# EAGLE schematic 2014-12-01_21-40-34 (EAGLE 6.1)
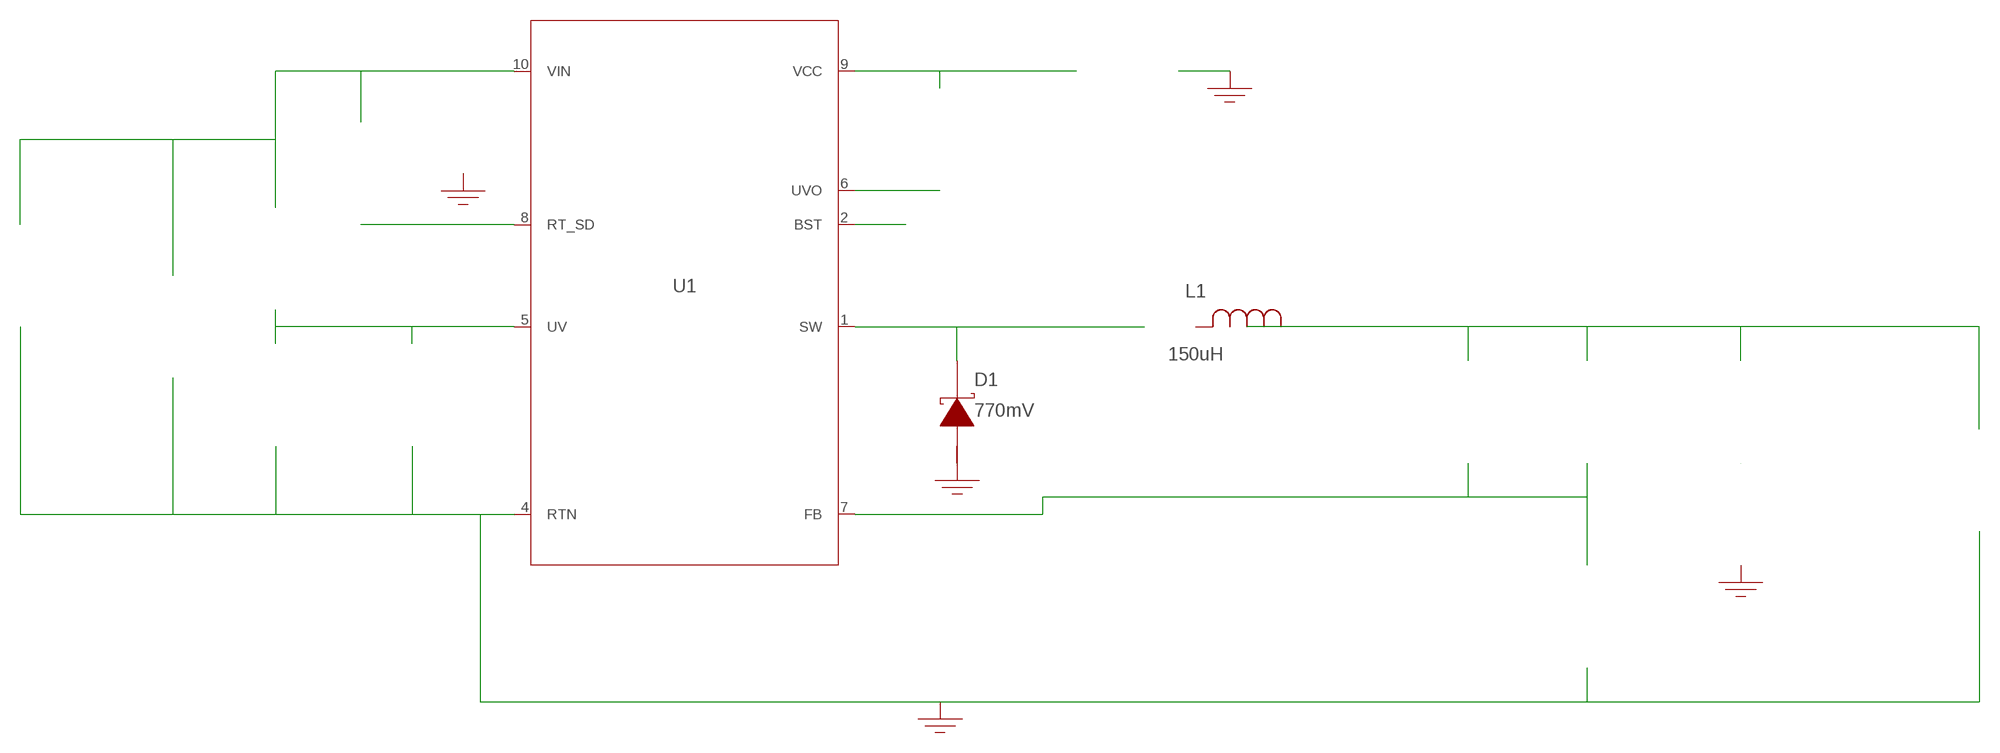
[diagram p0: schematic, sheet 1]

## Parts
CB  10nF  C1005X7R1C103KC1005X7R1C103K  [1005]  (not placed on a sheet)
CBYP  1uF  C1608X5R1C105KC1608X5R1C105K  [1608]  (not placed on a sheet)
CFF  2nF  GRM1885C1H202JA01DGRM1885C1H202JA01D  [0603]  (not placed on a sheet)
CIN  47uF  EEV-FK2A470QEEV-FK2A470Q  [SM_RADIAL_H13]  (not placed on a sheet)
CINX  100nF  C2012X7R2A104KC2012X7R2A104K  [0805]  (not placed on a sheet)
COUT  4.7uF  GRM21BR61C475KA88LGRM21BR61C475KA88L  [0805]  (not placed on a sheet)
CUV  1nF  GRM033R71E102KA01DGRM033R71E102KA01D  [0201]  (not placed on a sheet)
D1  770mV  DFLS1100-7DFLS1100-7  [PowerDI123]
GND  WB_GND  WB_GNDWB_GND  [WB_GND]
GND1  WB_GND  WB_GNDWB_GND  [WB_GND]
GND2  WB_GND  WB_GNDWB_GND  [WB_GND]
GND9999  WB_GND  WB_GNDWB_GND  [WB_GND]
GND_5  WB_GND  WB_GNDWB_GND  [WB_GND]
IOUT  WB_CURRENT_LOAD  WB_CURRENT_LOADWB_CURRENT_LOAD  [WB_CURRENT_LOAD]  (not placed on a sheet)
L1  150uH  CLF10040T-151MCLF10040T-151M  [CLF10040]
RFBB  3.32k  CRCW04023K32FKEDCRCW04023K32FKED  [0402]  (not placed on a sheet)
RFBT  10k  CRCW040210K0FKEDCRCW040210K0FKED  [0402]  (not placed on a sheet)
RON  178k  CRCW0402178KFKEDCRCW0402178KFKED  [0402]  (not placed on a sheet)
RSERIES  620m  ERJ-2BQFR62XERJ-2BQFR62X  [0402]  (not placed on a sheet)
RUV1  93.1k  CRCW040293K1FKEDCRCW040293K1FKED  [0402]  (not placed on a sheet)
RUV2  200k  CRCW0402200KFKEDCRCW0402200KFKED  [0402]  (not placed on a sheet)
RUVO  100k  CRCW0402100KFKEDCRCW0402100KFKED  [0402]  (not placed on a sheet)
U1  LM34923MM/NOPB  LM34923MM/NOPBLM34923MM/NOPB  [MUB10A]
VIN  WB_BATTERY  WB_BATTERYWB_BATTERY  [WB_BATTERY]  (not placed on a sheet)

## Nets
0: Cbyp.2@2 Cin.-@2 Cinx.2@2 Cuv.2@2 D1.2(A) GND1.1 GND2.1 GND9999.1 GND.1 GND_5.1 Iout.-@2 Rfbb.2@2 Rseries.2@2 Ruv1.2@2 U1.3(NC) U1.4(RTN) Vin.-@2
1: Cuv.1@1 Ruv1.1@1 Ruv2.2@2 U1.5(UV)
2: Cin.+@1 Cinx.1@1 Ron.1@1 Ruv2.1@1 U1.10(VIN) Vin.+@1
3: Cff.2@2 Rfbb.1@1 Rfbt.2@2 U1.7(FB)
4: Cb.2@2 D1.1(K) L1.1 U1.1(SW)
5: Cbyp.1@1 Ruvo.1@1 U1.9(VCC)
6: Cff.1@1 Cout.1@1 Iout.+@1 L1.2 Rfbt.1@1
7: Ron.2@2 U1.8(RT_SD)
8: Cb.1@1 U1.2(BST)
9: Ruvo.2@2 U1.6(UVO)
10: Cout.2@2 Rseries.1@1
Unconnected: CB.1 CB.2 CBYP.1 CBYP.2 CFF.1 CFF.2 CIN.1(+) CIN.2(-) CINX.1 CINX.2 COUT.1 COUT.2 CUV.1 CUV.2 IOUT.1(+) IOUT.2(-) RFBB.1 RFBB.2 RFBT.1 RFBT.2 RON.1 RON.2 RSERIES.1 RSERIES.2 RUV1.1 RUV1.2 RUV2.1 RUV2.2 RUVO.1 RUVO.2 VIN.1(+) VIN.2(-)

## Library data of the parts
CB = AcceleratedDesigns_Lib:C1005X7R1C103K; Cap: 1.0E-8; Datasheet_URL: http://www.tdk.co.jp/tefe02/e1688%5Fc.pdf; ESR: 0.072227; IRMS: 0.0; Manufacturer_Name: TDK; Manufacturer_Part_Number: C1005X7R1C103K; VDC: 16.0; Vendor: TDK
CBYP = AcceleratedDesigns_Lib:C1608X5R1C105K; Cap: 1.0E-6; Datasheet_URL: http://www.tdk.co.jp/tefe02/e2442%5Fc.pdf; ESR: 0.005713; IRMS: 0.0; Manufacturer_Name: TDK; Manufacturer_Part_Number: C1608X5R1C105K; VDC: 16.0; Vendor: TDK
CFF = AcceleratedDesigns_Lib:GRM1885C1H202JA01D; Cap: 2.0E-9; ESR: 0.0; IRMS: 0.0; Manufacturer_Name: MuRata; Manufacturer_Part_Number: GRM1885C1H202JA01D; VDC: 50.0; Vendor: MuRata
CIN = AcceleratedDesigns_Lib:EEV-FK2A470Q; Cap: 4.7E-5; Datasheet_URL: http://www.panasonic.com/industrial/components/pdf/smt%5Faec%5F050505.pdf; ESR: 0.32; IRMS: 0.5; Manufacturer_Name: Panasonic; Manufacturer_Part_Number: EEV-FK2A470Q; VDC: 100.0; Vendor: Panasonic
CINX = AcceleratedDesigns_Lib:C2012X7R2A104K; Cap: 1.0E-7; Datasheet_URL: http://www.tdk.co.jp/tefe02/e3555%5Fc.pdf; ESR: 0.015726; IRMS: 0.0; Manufacturer_Name: TDK; Manufacturer_Part_Number: C2012X7R2A104K; VDC: 100.0; Vendor: TDK
COUT = AcceleratedDesigns_Lib:GRM21BR61C475KA88L; Cap: 4.7E-6; ESR: 0.0050; IRMS: 0.0; Manufacturer_Name: MuRata; Manufacturer_Part_Number: GRM21BR61C475KA88L; VDC: 16.0; Vendor: MuRata
CUV = AcceleratedDesigns_Lib:GRM033R71E102KA01D; Cap: 1.0E-9; ESR: 0.0; IRMS: 0.0; Manufacturer_Name: MuRata; Manufacturer_Part_Number: GRM033R71E102KA01D; VDC: 25.0; Vendor: MuRata
D1 = AcceleratedDesigns_Lib:DFLS1100-7; Datasheet_URL: http://www.diodes.com/datasheets/ds30497.pdf; Io: 1.0; Manufacturer_Name: Diodes Inc.; Manufacturer_Part_Number: DFLS1100-7; VFatIo: 0.77; VRRM: 100.0; Vendor: Diodes Inc.
GND GND1 GND2 GND9999 GND_5 = AcceleratedDesigns_Lib:WB_GND; Manufacturer_Name: WB_GND; Manufacturer_Part_Number: WB_GND; PowerPortType: POWER_GROUND; Value: Value
IOUT = AcceleratedDesigns_Lib:WB_CURRENT_LOAD; Manufacturer_Name: WB_CURRENT_LOAD; Manufacturer_Part_Number: WB_CURRENT_LOAD; PowerPortType: POWER_GROUND; Value: Value
L1 = AcceleratedDesigns_Lib:CLF10040T-151M; Manufacturer_Name: TDK; Manufacturer_Part_Number: 'CLF10040T-151M'; Vendor: Gimme a name
RFBB = AcceleratedDesigns_Lib:CRCW04023K32FKED; Manufacturer_Name: Vishay-Dale; Manufacturer_Part_Number: CRCW04023K32FKED; Power: 0.063; Resistance: 3320.0; Tolerance: 1.0; Vendor: Vishay-Dale
RFBT = AcceleratedDesigns_Lib:CRCW040210K0FKED; Manufacturer_Name: Vishay-Dale; Manufacturer_Part_Number: CRCW040210K0FKED; Power: 0.063; Resistance: 10000.0; Tolerance: 1.0; Vendor: Vishay-Dale
RON = AcceleratedDesigns_Lib:CRCW0402178KFKED; Manufacturer_Name: Vishay-Dale; Manufacturer_Part_Number: CRCW0402178KFKED; Power: 0.063; Resistance: 178000.0; Tolerance: 1.0; Vendor: Vishay-Dale
RSERIES = AcceleratedDesigns_Lib:ERJ-2BQFR62X; Manufacturer_Name: Panasonic; Manufacturer_Part_Number: ERJ-2BQFR62X; Power: 0.125; Resistance: 0.62; Tolerance: 1.0; Vendor: Panasonic
RUV1 = AcceleratedDesigns_Lib:CRCW040293K1FKED; Manufacturer_Name: Vishay-Dale; Manufacturer_Part_Number: CRCW040293K1FKED; Power: 0.063; Resistance: 93100.0; Tolerance: 1.0; Vendor: Vishay-Dale
RUV2 = AcceleratedDesigns_Lib:CRCW0402200KFKED; Manufacturer_Name: Vishay-Dale; Manufacturer_Part_Number: CRCW0402200KFKED; Power: 0.063; Resistance: 200000.0; Tolerance: 1.0; Vendor: Vishay-Dale
RUVO = AcceleratedDesigns_Lib:CRCW0402100KFKED; Manufacturer_Name: Vishay-Dale; Manufacturer_Part_Number: CRCW0402100KFKED; Power: 0.063; Resistance: 100000.0; Tolerance: 1.0; Vendor: Vishay-Dale
U1 = AcceleratedDesigns_Lib:LM34923MM/NOPB; Datasheet_URL: http://www.ti.com/product/lm34923; Frequency: 800000.0; Imax: 0.6; Manufacturer_Name: Texas Instruments; Manufacturer_Part_Number: LM34923MM/NOPB; Mktg_Package: NA; NSID: LM34923MM/NOPB; Package: NA; Vendor: Texas Instruments
VIN = AcceleratedDesigns_Lib:WB_BATTERY; Manufacturer_Name: WB_BATTERY; Manufacturer_Part_Number: WB_BATTERY; PowerPortType: POWER_GROUND; Value: Value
